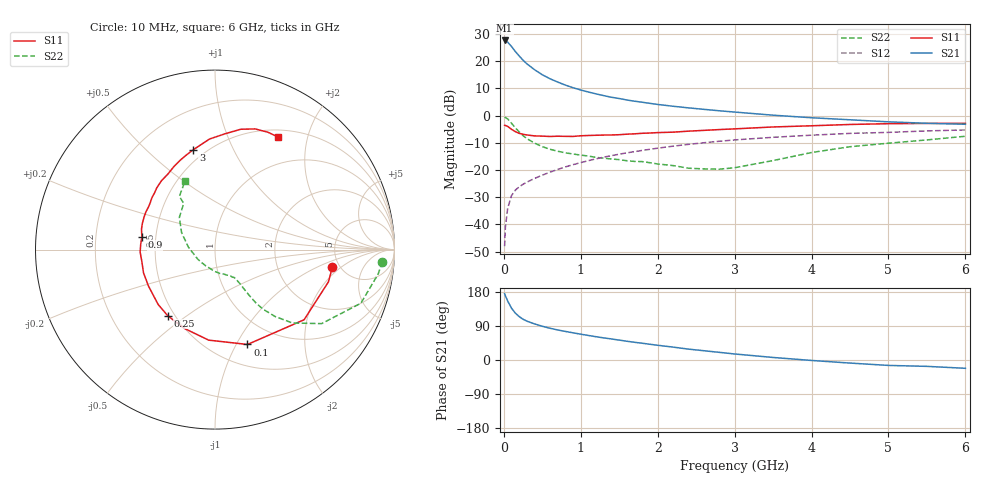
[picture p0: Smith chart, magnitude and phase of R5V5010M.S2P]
! SIEMENS Small Signal Semiconductors
! BFR183
! Si NPN RF Bipolar Junction Transistor in SOT23
! VCE = 0.5 V  IC = 10 mA
! Common Emitter S-Parameters:  May  1996
# GHz  S  MA  R  50
!  f  S11  S21  S12  S22
! GHz  MAG  ANG  MAG  ANG  MAG  ANG  MAG  ANG
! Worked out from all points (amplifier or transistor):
!   36 points, 10 MHz to 6 GHz, reference 50 ohm
!   highest |S21| = 27.6 dB at 10 MHz (marker M1)
!   |S21| within 3 dB of that: start of sweep to 121.1 MHz
!   unconditionally stable (mu >= 1): 562.9 MHz to 4.103 GHz; 5.942 GHz to end of sweep
!   at 250 MHz: K = 0.68, MSG = 22.8 dB, |S12| = -25.2 dB
!   at 1.4 GHz: K = 1.12, MAG = 8.6 dB, |S12| = -14.7 dB
!   at 6 GHz: K = 1.00, MAG = 0.8 dB, |S12| = -5.3 dB
!   S11 on the Smith chart (normalised r, x): 10 MHz: 4.37, -1.50; 100 MHz: 0.72, -1.11; 250 MHz: 0.46, -0.43; 900 MHz: 0.42, +0.07; 3 GHz: 0.43, +0.71; 6 GHz: 0.59, +1.54
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0.01  0.6616 -8.4  23.9 175.0  0.004 84.6  0.9343 -4.2
0.02  0.657 -15.9  23.6 169.6  0.0089 82.4  0.9194 -8.5
0.05  0.6319 -38.2  22.23 155.6  0.0199 73.3  0.8659 -20.2
0.1  0.5587 -71.1  18.51 136.8  0.034 61.7  0.7229 -34.8
0.15  0.5057 -94.0  14.96 123.6  0.0428 57.1  0.5937 -43.5
0.2  0.4708 -111.6  12.39 114.5  0.0493 54.5  0.5004 -48.1
0.25  0.4528 -125.6  10.36 107.5  0.0547 53.8  0.4264 -51.1
0.3  0.4402 -136.0  8.892 102.5  0.06 54.7  0.3762 -52.5
0.4  0.4227 -151.1  6.932 95.2  0.0701 55.8  0.3117 -53.3
0.5  0.4188 -162.0  5.608 89.0  0.0805 57.0  0.2686 -53.6
0.6  0.4129 -170.9  4.734 83.8  0.0912 58.1  0.2404 -53.7
0.7  0.4173 -178.1  4.118 79.3  0.1025 58.7  0.2214 -54.1
0.9  0.4136 170.2  3.243 71.7  0.1255 58.9  0.1968 -54.8
1.1  0.4304 160.0  2.699 64.7  0.1486 58.4  0.1803 -57.9
1.3  0.4384 151.6  2.318 58.3  0.1724 57.0  0.1645 -61.1
1.6  0.455 140.6  1.928 49.5  0.2068 54.2  0.1481 -68.7
2.2  0.4953 122.2  1.481 34.0  0.2741 47.3  0.1206 -92.2
3  0.5693 102.3  1.159 15.9  0.3568 36.3  0.1101 -151.4
3.5  0.617 92.8  1.015 6.7  0.3987 29.1  0.1491 174.6
4.5  0.6858 77.9  0.836 -8.1  0.4703 15.6  0.2678 137.9
5.5  0.7173 65.8  0.721 -16.8  0.5224 4.4  0.3568 123.8
6  0.719 60.8  0.692 -21.9  0.544 -2.9  0.4167 113.6
